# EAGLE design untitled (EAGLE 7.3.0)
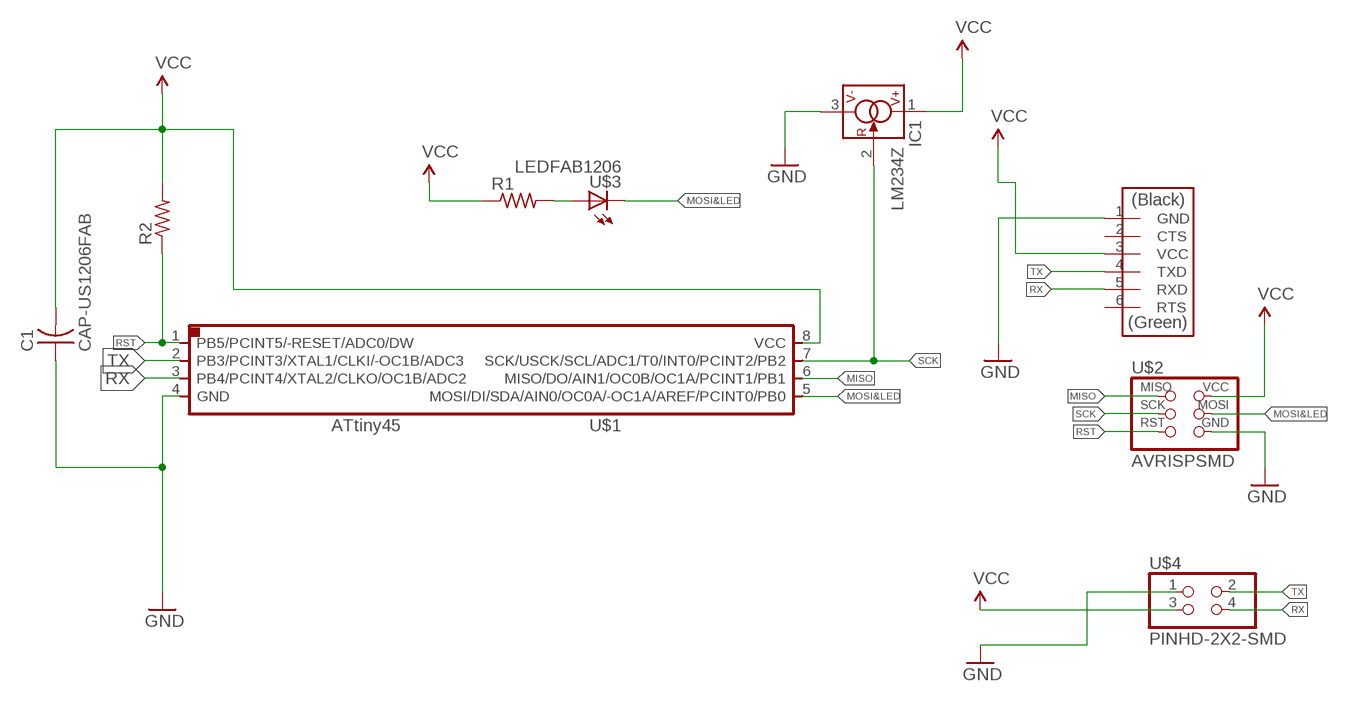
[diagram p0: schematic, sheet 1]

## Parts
C1  CAP-US1206FAB  [C1206FAB]
IC1  LM234Z  [TO92]
R1  RES-US1206FAB  [R1206FAB]
R2  RES-US1206FAB  [R1206FAB]
U$1  ATTINY45SI  [SOIC8]
U$2  AVRISPSMD  [2X03SMD]
U$3  LEDFAB1206  [LED1206FAB]
U$4  PINHD-2X2-SMD  [2X02SMD]
U$5  FTDI-SMD-HEADER  [1X06SMD]

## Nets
GND: C1.1 IC1.3(V-) U$1.4(GND) U$2.6(GND) U$4.1 U$5.1(GND)
MISO: U$1.6(MISO/DO/AIN1/OC0B/OC1A/PCINT1/PB1) U$2.1(MISO)
MOSI&LED: U$1.5(MOSI/DI/SDA/AIN0/OC0A/-OC1A/AREF/PCINT0/PB0) U$2.4(MOSI) U$3.2(C)
N$2: R1.2 U$3.1(A)
RST: R2.1 U$1.1(PB5/PCINT5/-RESET/ADC0/DW) U$2.5(RST)
RX: U$1.3(PB4/PCINT4/XTAL2/CLKO/OC1B/ADC2) U$4.4 U$5.5(RXD)
SCK: IC1.2(R) U$1.7(SCK/USCK/SCL/ADC1/T0/INT0/PCINT2/PB2) U$2.3(SCK)
TX: U$1.2(PB3/PCINT3/XTAL1/CLKI/-OC1B/ADC3) U$4.2 U$5.4(TXD)
VCC: C1.2 IC1.1(V+) R1.1 R2.2 U$1.8(VCC) U$2.2(VCC) U$4.3 U$5.3(VCC)
Unconnected: U$5.2(CTS) U$5.6(RTS)

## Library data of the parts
C1 = fab:CAP-US
IC1 = linear:LM*34: 3-Terminal Adjustable Current Sources Source: www.national.com/pf/LM/LM334.html | LM134.pdf
R1 R2 = fab:RES-US: Resistor (US Symbol)
U$1 = fab:ATTINY45
U$2 = fab:AVRISP
U$3 = fab:LED: LED
U$4 = fab:PINHD-2X2-SMD
U$5 = fab:FTDI-SMD-HEADER

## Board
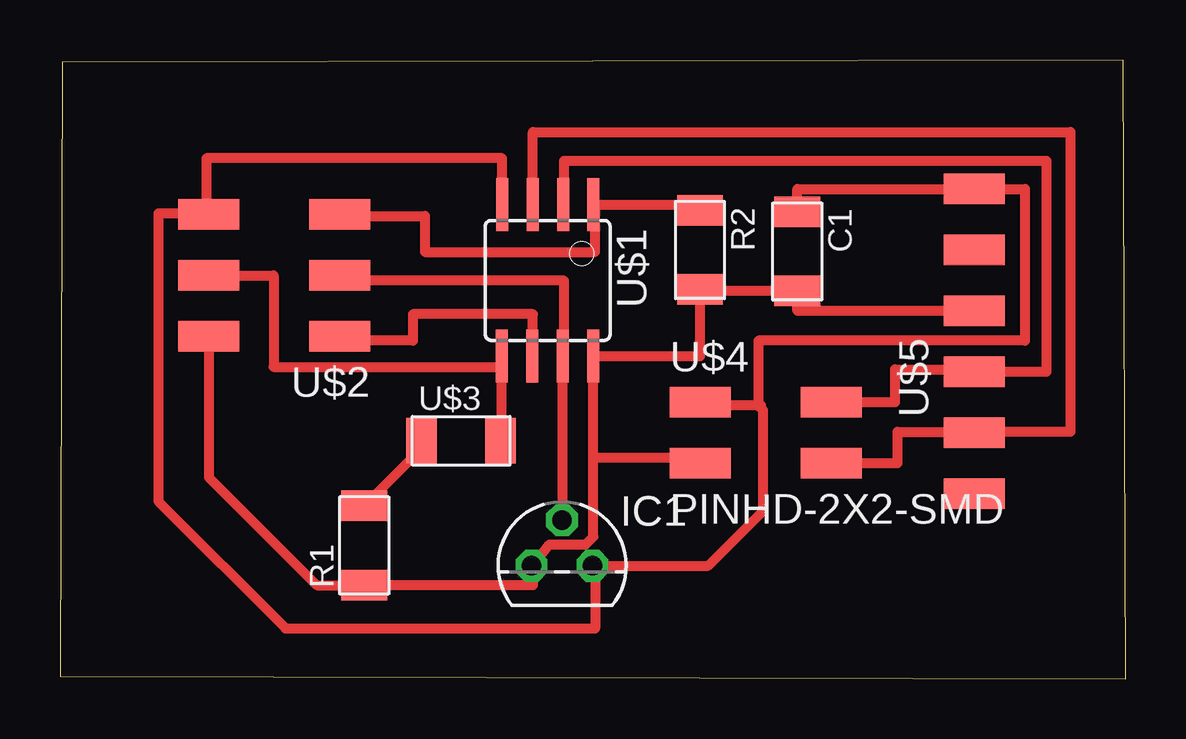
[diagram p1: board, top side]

Size 44.4 x 25.8 mm. Coordinates in mm from the lower left corner, seen from the top.
Outline: 0,0.1 44.4,0 44.3,25.8 0.1,25.7 0,0.1
Copper layers (1*16): Top 0.035mm / dielectric 1.5mm / Bottom 0.035mm
Design rules "default": minimum track width 10mil, minimum drill 24mil, track to track 8mil, track to pad 8mil, pad to pad 8mil, via to via 8mil, smd to smd 8mil, copper to edge 40mil, drill to drill 8mil, minimum pad ring 10mil, minimum via ring 8mil, stop-mask expansion 4mil, vias tented up to drill 0mil, thermal gap 10mil

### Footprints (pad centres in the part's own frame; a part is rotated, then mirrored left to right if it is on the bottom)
C1206FAB = smd 1.27 x 1.905: 1 -1.651,0; 2 1.651,0
TO92 = drill 0.813 octagon: 1 -1.27,0; 2 0,1.905; 3 1.27,0
R1206FAB = smd 1.27 x 1.905: 1 -1.651,0; 2 1.651,0
SOIC8 = smd 0.5 x 2.2: 1 -1.905,-3.154; 2 -0.645,-3.154; 3 0.625,-3.154; 4 1.895,-3.154; 5 1.905,3.154; 6 0.635,3.154; 7 -0.635,3.154; 8 -1.905,3.154
2X03SMD = smd 2.54 x 1.27: 1 -2.54,2.54; 2 2.92,2.54; 3 -2.54,0; 4 2.92,0; 5 -2.54,-2.54; 6 2.92,-2.54
LED1206FAB = smd 1.27 x 1.905: 1 -1.651,0; 2 1.651,0
2X02SMD = smd 2.54 x 1.27: 1 -2.54,1.27; 2 2.92,1.27; 3 -2.54,-1.27; 4 2.92,-1.27
1X06SMD = smd 2.54 x 1.27: 1 0,6.35; 2 0,3.81; 3 0,1.27; 4 0,-1.27; 5 0,-3.81; 6 0,-6.35

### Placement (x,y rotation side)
C1  30.72,17.82 270 top
IC1  20.92,4.71 0 top
R1  12.68,5.56 90 top
R2  26.67,17.88 270 top
U$1  20.32,16.61 180 top
U$2  9.12,16.82 180 top
U$3  16.71,9.92 0 top
U$4  29.21,10.26 0 top
U$5  38.1,14.07 0 top

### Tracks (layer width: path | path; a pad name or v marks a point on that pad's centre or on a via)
GND
  Top 0.406: 29.1,11.4 29.1,14.1 40.2,14.1 40.2,20.42 U$5.1 30.72,20.42 C1.1 | 29.1,11.4 26.67,11.4 U$4.1 | 29.2,11.4 29.1,11.4 | U$1.4 18.43,21.7 6.1,21.7 6.1,19.36 U$2.6 6.2,19.4 4.1,19.4 4.1,7.4 9.4,2.1 22.3,2.1 22.3,4.71 | IC1.3 22.3,4.71 | 22.3,4.71 27.01,4.71 29.3,7 29.3,11.2 29.1,11.4
MISO
  Top 0.406: U$1.6 19.7,13.46 19.7,15.2 14.7,15.2 14.7,14.1 11.66,14.1 U$2.1
MOSI&LED
  Top 0.406: U$3.2 18.41,9.92 U$1.5 18.41,13 8.9,13 8.9,16.82 U$2.4
N$2
  Top 0.406: U$3.1 15.06,9.59 R1.2
RST
  Top 0.406: R2.1 26.67,19.76 U$1.1 22.3,19.76 22.3,17.8 15.2,17.8 15.2,19.3 11.66,19.3 U$2.5
RX
  Top 0.406: U$4.4 34.9,8.99 34.9,10.3 38.1,10.3 | U$1.3 19.7,22.8 42.1,22.8 42.1,10.3 38.1,10.3 | 38.1,10.3 U$5.5
SCK
  Top 0.406: U$1.7 20.9,13.46 | U$1.7 21,13.46 21,16.6 11.66,16.6 U$2.3 | U$1.7 20.92,13.46 IC1.2
TX
  Top 0.406: U$4.2 34.8,11.53 34.8,12.9 38.1,12.9 U$5.4 41.1,12.8 41.1,21.6 21,21.6 21,19.76 U$1.2
VCC
  Top 0.406: U$4.3 26.5,8.99 26.5,9.2 22.23,9.2 | U$5.3 30.72,15.34 C1.2 26.67,16.17 R2.2 26.67,13.46 U$1.8 22.23,9.2 | IC1.1 19.7,4.71 | 19.7,4.71 19.7,3.91 R1.1 10.7,3.9 6.2,8.4 U$2.2 | 19.7,4.71 20.39,5.6 21.9,5.6 22.23,5.92 22.23,9.2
